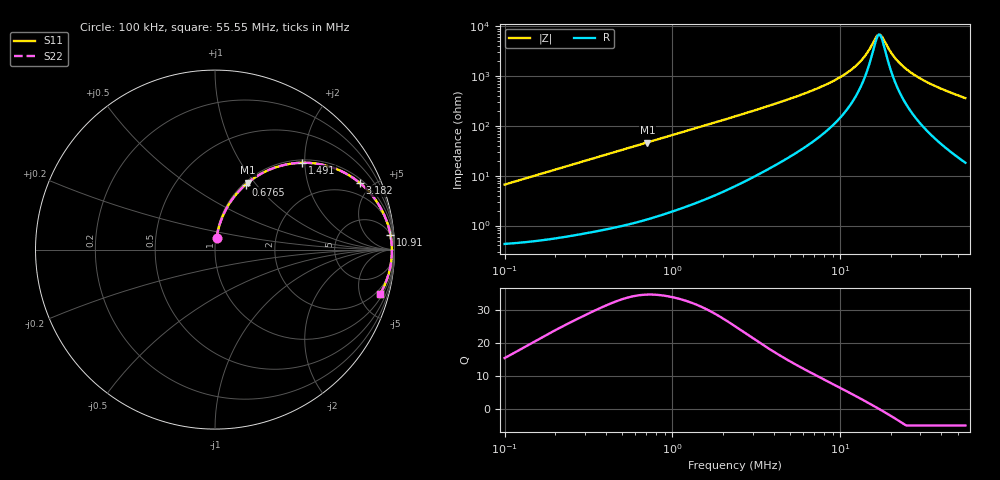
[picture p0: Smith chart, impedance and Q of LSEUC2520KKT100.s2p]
! LSEUC2520KKT100  S-PARAMETER MODEL  ( General Type )
! Model Generated by TAIYO YUDEN Corporation (http://www.ty-top.com)
! Version 1.0
! TAIYO YUDEN Control No. 220210
! Copyright(c) 2022 TAIYO YUDEN CO.,LTD. All Rights Reserved.
! Product Description (link to TY-COMPAS)
! https://ds.yuden.co.jp/TYCOMPAS/or/detail?pn=LSEUC2520KKT100M&u=M
! Products Name : Inductors
! Characteristics :
!  Inductance : 10 uH , SRF(min) : -Hz , DC Resistance(max) : 0.432 Ohm
!  Rated Current : Saturation :1000 mA , Temp Rise : 1000 mA (40 degC)
!  Case Size : 2.5 x 2.0 / 0.098 x 0.079 [mm/inch] , Thickness : 1 / 0.039 [mm/inch]
!  (Conditions: Temperature = 25 degC , DC Bias Current/Voltage = 0A / 0V)
! External Node Assignments :
!  1  o---GGG---o  2
! GND o---------o GND
! Frequency Range : 0.1MHz  -  55.545741MHz  [ 402 STEP ]
# MHz S RI R 50
! Freq[MHz].  S11 Real  S11 Imag  S21 Real  S21 Imag  S12 Real  S12 Imag  S22 Real  S22 Imag
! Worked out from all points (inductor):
!   401 points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, 100 kHz to 55.55 MHz, reference 50 ohm
!   read as one part in series: L = 10.6 uH near 103.2 kHz
!   highest Q = 34.8 at 709.3 kHz (marker M1), where L = 10.4 uH
!   self-resonance near 16.98 MHz
!   S11 on the Smith chart (normalised r, x): 100 kHz: 1.01, +0.13; 676.5 kHz: 1.03, +0.88; 1.491 MHz: 1.06, +1.95; 3.182 MHz: 1.20, +4.24; 10.91 MHz: 5, +23; 55.55 MHz: 1.36, -7.23
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0.1  0.0086 0.0655  0.9914 -0.0655  0.9914 -0.0655  0.0086 0.0655
0.288223  0.0408 0.1809  0.9592 -0.1809  0.9592 -0.1809  0.0408 0.1809
0.455739  0.089 0.2698  0.911 -0.2698  0.911 -0.2698  0.089 0.2698
0.676483  0.1708 0.3622  0.8292 -0.3622  0.8292 -0.3622  0.1708 0.3622
0.709319  0.184 0.3734  0.816 -0.3734  0.816 -0.3734  0.184 0.3734
0.830726  0.234 0.4092  0.766 -0.4092  0.766 -0.4092  0.234 0.4092
1.490521  0.4871 0.484  0.5129 -0.484  0.5129 -0.484  0.4871 0.484
2.394347  0.7057 0.4361  0.2943 -0.4361  0.2943 -0.4361  0.7057 0.4361
3.181972  0.8069 0.3714  0.1931 -0.3714  0.1931 -0.3714  0.8069 0.3714
4.504557  0.8915 0.2811  0.1085 -0.2811  0.1085 -0.2811  0.8915 0.2811
6.792887  0.948 0.1807  0.052 -0.1807  0.052 -0.1807  0.948 0.1807
8.885913  0.9681 0.1227  0.0319 -0.1227  0.0319 -0.1227  0.9681 0.1227
10.91197  0.9776 0.082  0.0224 -0.082  0.0224 -0.082  0.9776 0.082
12.38215  0.9814 0.0581  0.0186 -0.0581  0.0186 -0.0581  0.9814 0.0581
13.61338  0.9835 0.0406  0.0165 -0.0406  0.0165 -0.0406  0.9835 0.0406
16.71734  0.9856 0.00329  0.0144 -0.00329  0.0144 -0.00329  0.9856 0.00329
17.52879  0.9856 -0.00528  0.0144 0.00528  0.0144 0.00528  0.9856 -0.00528
19.57868  0.9852 -0.0254  0.0148 0.0254  0.0148 0.0254  0.9852 -0.0254
22.92977  0.983 -0.0546  0.017 0.0546  0.017 0.0546  0.983 -0.0546
28.15793  0.9771 -0.0943  0.0229 0.0943  0.0229 0.0943  0.9771 -0.0943
38.01646  0.9604 -0.1578  0.0396 0.1578  0.0396 0.1578  0.9604 -0.1578
55.54574  0.9183 -0.2499  0.0817 0.2499  0.0817 0.2499  0.9183 -0.2499
